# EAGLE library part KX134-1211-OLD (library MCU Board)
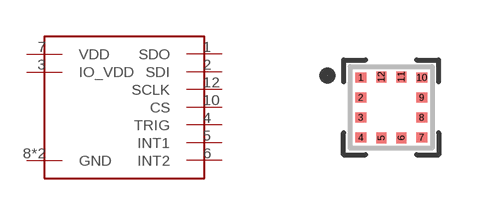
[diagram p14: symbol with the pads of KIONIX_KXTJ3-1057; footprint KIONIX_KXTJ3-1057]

Designator prefix U

## KX134-1211-OLD  [KIONIX_KXTJ3-1057]
1  SDO
2  SDI
3  IO_VDD
4  TRIG
5  INT1
6  INT2
7  VDD
8  GND
9  GND
10  CS
12  SCLK

## Footprint KIONIX_KXTJ3-1057 (pad centres in mm)
smd 0.275 x 0.25: 1 -0.762,0.75; 2 -0.762,0.25; 3 -0.762,-0.25; 4 -0.762,-0.75; 7 0.762,-0.75; 8 0.762,-0.25; 9 0.762,0.25; 10 0.762,0.75
smd 0.25 x 0.275: 5 -0.25,-0.762; 6 0.25,-0.762; 11 0.25,0.762; 12 -0.25,0.762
